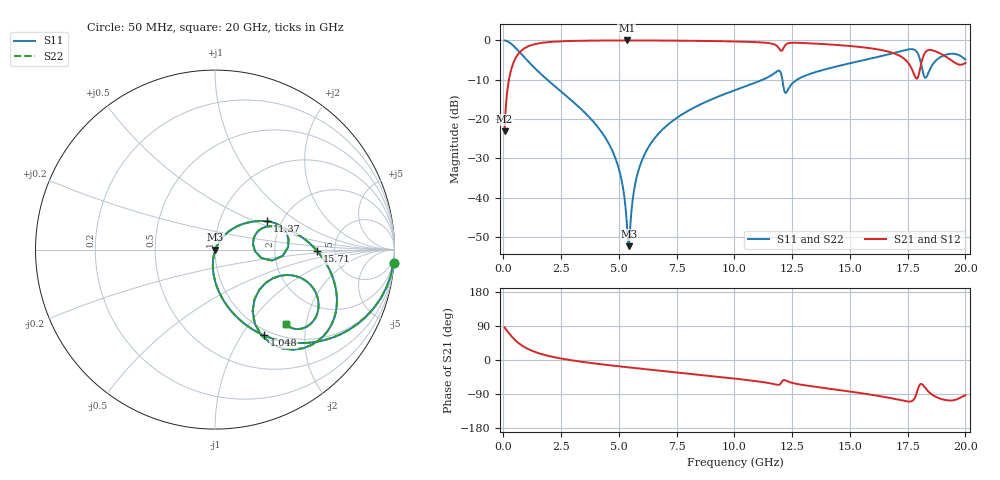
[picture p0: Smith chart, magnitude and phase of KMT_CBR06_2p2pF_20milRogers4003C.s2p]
! Data measured by Modelithics Inc. support@modelithics.com 813-866-6335
! KEMET CBR0603 2.2pF, Pad Width= 0.851mm, Pad Length= 0.64mm, Pad Gap= 0.62mm, 20mil Rogers 4003C substrate Data, January 2022
# hz S ma R 50
! 2 Port Network Data from SP1.SP block
! freq  magS11  angS11  magS21  angS21  magS12  angS12  magS22  angS22
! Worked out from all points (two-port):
!   401 points, 50 MHz to 20 GHz, reference 50 ohm
!   highest |S21| = -0.02 dB at 5.337 GHz (marker M1); lowest = -23.1 dB at 50 MHz (marker M2)
!   |S21| within 3 dB of the highest: 703 MHz to 16.77 GHz (16.06 GHz wide, 184 % of centre); 18.27 GHz to 18.8 GHz (530 MHz wide, 2.86 % of centre)
!   lowest |S11| = -52.3 dB at 5.436 GHz (marker M3), VSWR 1.00, Z = 50.2 + j0.00361 ohm
!   |S11| at or under -10 dB: 1.898 GHz to 11.22 GHz (9.322 GHz wide, 142 % of centre); 12.08 GHz to 12.71 GHz (633.7 MHz wide, 5.11 % of centre)
!   |S22| runs from -52.3 to 0.0 dB; largest |S21 - S12| = 0
!   S11 on the Smith chart (normalised r, x): 50 MHz: 1, -27; 1.048 GHz: 0.92, -1.26; 11.37 GHz: 1.69, +0.60; 15.71 GHz: 3.66, -0.11; 20 GHz: 1.25, -1.53
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5e7  0.9975 -4.2  0.06985 85.8  0.06985 85.8  0.9975 -4.2
3.99125e8  0.8714 -30.7  0.4894 59.2  0.4894 59.2  0.8714 -30.7
1.0475e9  0.5494 -60.3  0.8342 29.5  0.8342 29.5  0.5494 -60.3
3.391625e9  0.1315 -93.9  0.9893 -4.7  0.9893 -4.7  0.1315 -93.9
4.788125e9  0.03522 -101.7  0.9971 -15.2  0.9971 -15.2  0.03522 -101.7
5.13725e9  0.01551 -99.4  0.9975 -17.6  0.9975 -17.6  0.01551 -99.4
5.33675e9  0.00502 -82.2  0.9975 -18.9  0.9975 -18.9  0.00502 -82.2
5.4365e9  0.002429 0.8  0.9975 -19.6  0.9975 -19.6  0.002429 0.8
5.885375e9  0.02428 61.9  0.9971 -22.5  0.9971 -22.5  0.02428 61.9
6.73325e9  0.06623 59.9  0.995 -27.9  0.995 -27.9  0.06623 59.9
1.0025e10  0.2332 39.9  0.9681 -49.1  0.9681 -49.1  0.2332 39.9
1.137162e10  0.3312 28.4  0.9317 -59.6  0.9317 -59.6  0.3312 28.4
1.192025e10  0.4138 8.2  0.8012 -65.5  0.8012 -65.5  0.4138 8.2
1.226938e10  0.2223 15.1  0.9032 -55.4  0.9032 -55.4  0.2223 15.1
1.336662e10  0.383 19.2  0.9144 -69.5  0.9144 -69.5  0.383 19.2
1.571075e10  0.5711 -1.0  0.8066 -89.6  0.8066 -89.6  0.5711 -1.0
1.670825e10  0.6679 -12.5  0.7139 -99.9  0.7139 -99.9  0.6679 -12.5
1.7606e10  0.7726 -33.3  0.4766 -109.6  0.4766 -109.6  0.7726 -33.3
1.790525e10  0.709 -51.8  0.3258 -84.3  0.3258 -84.3  0.709 -51.8
1.815462e10  0.4012 -58.5  0.6 -65.5  0.6 -65.5  0.4012 -58.5
1.90025e10  0.6317 -25.1  0.6592 -103.7  0.6592 -103.7  0.6317 -25.1
2e10  0.5707 -46.4  0.5176 -93.2  0.5176 -93.2  0.5707 -46.4
